| IBIS file 70t3519z.ibs created by s2ibis2 version 1.1
| North Carolina State University Electronics Research Laboratory  1995
[IBIS ver]   2.1
[File name]   70t3519bf.ibs
[File Rev]   3.0
|1.0 : Original Version - Wei-Ling Chang
|2.0 : Corrected Ramp rates and package RLC values - Wei-Ling Chang
|3.0 : Replaced I/O and Input models with ADC models - Sunil Kashyap
[Date]   03/30/04
[Disclaimer] Integrated Device Technology, Inc. ("IDT") hereby grants the
   user of this IBIS model a non-exclusive, nontransferable
   license to use this IBIS model under the following terms. The
   user is granted this license only to use the IBIS model and is
   not granted rights to sell, copy (except as needed to run the
   IBIS model), rent, lease or sub-license the IBIS model in
   whole or in part, or in modified form to anyone. The User may
   modify the IBIS model to suit its specific applications, but
   rights to derivative works and such modifications shall belong
   to IDT. This IBIS model is provided on an AS IS" basis and IDT
   makes absolutely no warranty with respect to the information
   contained herein. IDT DISCLAIMS AND CUSTOMER WAIVES ALL
   WARRANTIES, EXPRESS AND IMPLIED, INCLUDING WARRANTIES OF
   MERCHANTABILITY AND FITNESS FOR A PARTICULAR PURPOSE. THE
   ENTIRE RISK AS TO QUALITY AND PERFORMANCE IS WITH THE USER
   ACCORDINGLY, IN NO EVENT SHALL IDT BE LIABLE FOR ANY DIRECT OR
   INDIRECT DAMAGES, WHETHER IN CONTRACT OR TORT, INCLUDING ANY
   LOST PROFITS OR OTHER INCIDENTAL, CONSEQUENTIAL, EXEMPLARY, OR
   PUNITIVE DAMAGES ARISING OUT OF THE USE OR APPLICATION OF THE
   IBIS model. Further, IDT reserves the right to make changes
   without notice to any product herein to improve reliability,
   function, or design. IDT does not convey any license under
   patent rights or any other intellectual property rights,
   including those of third parties. IDT is not obligated to
   provide maintenance or support for the licensed IBIS model.
[Copyright]   Copyright 2001, Integrated Device Technology, Inc. all rights
   reserved
|   Component 70t3519z
[Component]   70t3519z
[Manufacturer]   Integrated Device Technology
[Package]
|208-pin fpBGA
| variable   typ   min   max
R_pkg   0.10000   0.05000   0.30000
L_pkg   12.0000nH   10.0000nH   14.00000nH
C_pkg   2.80000pF   1.50000pF   6.00000pF
| NOTE:
| The model_name inpad25, inpadzz25, inpadbs25, and iopad25 work for both
| 3.3v and 2.5v vddq.  When vddq is 3.3v, the model names are inpad33,
| inpadzz33, inpadbs33, and iopad33.  When vddq is 2.5v, the model names
| will be inpad25, inpadzz25, inpadbs25, and iopad25.
[Pin]  signal_name   model_name   R_pin   L_pin   C_pin
A1   io19l   iopad25
C2   io19r   iopad25
D4   io20l   iopad25
B1   io20r   iopad25
C1   vddql   POWER
A3   vss/test   GND
D3   io21l   iopad25
E4   io21r   iopad25
D1   io22l   iopad25
E2   io22r   iopad25
C3   vddqr   POWER
A17   vss   GND
E1   io23l   iopad25
F2   io23r   iopad25
F3   io24l   iopad25
G4   io24r   iopad25
F1   vddql   POWER
B2   vss   GND
G3   io25l   iopad25
H4   io25r   iopad25
G1   io26l   iopad25
H2   io26r   iopad25
E3   vddqr   POWER
B10   vss   GND
H1   vdd   POWER
J2   vdd   POWER
C10   vss   GND
J1   vddql   POWER
J4   zzr   inpadzz25
K3   io27r   iopad25
L4   io27l   iopad25
K1   io28r   iopad25
L2   io28l   iopad25
H3   vddqr   POWER
C17   vss   GND
L1   io29r   iopad25
M2   io29l   iopad25
M3   io30r   iopad25
N4   io30l   iopad25
M1   vddql   POWER
D2   vss   GND
N3   io31r   iopad25
N1   io31l   iopad25
P1   io32r   iopad25
P2   io32l   iopad25
L3   vddqr   POWER
E16   vss   GND
T1   io33r   iopad25
R2   io33l   iopad25
R3   io34r   iopad25
T2   io34l   iopad25
F4   vss   GND
T3   vddql   POWER
P4   io35r   iopad25
U2   io35l   iopad25
U3   plftr#   inpad25
U4   colr#   iopad25
T4   tms   inpadbs25
R4   tck   inpadbs25
P5   trstb   inpadbs25
T5   intr#   iopad25
R5   a17r   inpad25
P6   a16r   inpad25
U5   a15r   inpad25
T6   a14r   inpad25
R6   a13r   inpad25
P7   a12r   inpad25
U6   a11r   inpad25
T7   a10r   inpad25
R7   a9r   inpad25
P8   a8r   inpad25
U7   a7r   inpad25
T8   be3rb   inpad25
R8   be2rb   inpad25
P9   be1rb   inpad25
U8   be0rb   inpad25
T9   ce1r   inpad25
R9   ce0r   inpad25
C4   plftl#   inpad25
D9   vdd   POWER
F14   vss   GND
G2   vss   GND
P11   clkr#   inpad25
U10   oerb   inpad25
T11   rwrb   inpad25
R11   adsr#   inpad25
P12   cntenr#   inpad25
U11   repeatr#   inpad25
T12   a6r   inpad25
R12   a5r   inpad25
P13   a4r   inpad25
U12   a3r   inpad25
T13   a2r   inpad25
R13   a1r   inpad25
U13   a0r   inpad25
U9   vdd   POWER
H16   vss   GND
J3   vss   GND
U15   optr   inpad25
U16   io0l   iopad25
T15   io0r   iopad25
R15   vddql   POWER
J16   vss   GND
U17   io1l   iopad25
R16   io1r   iopad25
P14   io2l   iopad25
T17   io2r   iopad25
P3   vddqr   POWER
K2   vss   GND
P15   io3l   iopad25
N14   io3r   iopad25
P17   io4l   iopad25
N16   io4r   iopad25
N15   vddql   POWER
K4   vss   GND
N17   io5l   iopad25
M16   io5r   iopad25
M15   io6l   iopad25
L14   io6r   iopad25
R17   vddqr   POWER
K17   vss   GND
L15   io7l   iopad25
K14   io7r   iopad25
L17   io8l   iopad25
K16   io8r   iopad25
K15   vddql   POWER
L16   vss   GND
M4   vss   GND
M14   vss   GND
A10   vdd   POWER
P10   vdd   POWER
M17   vddqr   POWER
N2   vss   GND
H15   io9r   iopad25
G14   io9l   iopad25
H17   io10r   iopad25
G16   io10l   iopad25
G15   vddql   POWER
P16   vss   GND
G17   io11r   iopad25
F16   io11l   iopad25
F15   io12r   iopad25
E14   io12l   iopad25
J17   vddqr   POWER
R1   vss   GND
E15   io13r   iopad25
E17   io13l   iopad25
D17   io14r   iopad25
D16   io14l   iopad25
D15   vddql   POWER
J14   zzl   inpadzz25
B17   io15r   iopad25
C16   io15l   iopad25
C15   io16r   iopad25
B16   io16l   iopad25
R10   vss   GND
F17   vddqr   POWER
D14   io17r   iopad25
A16   io17l   iopad25
A15   optl   inpad25
D13   vdd   POWER
C14   vdd   POWER
A14   a0l   inpad25
B13   a1l   inpad25
C13   a2l   inpad25
D12   a3l   inpad25
A13   a4l   inpad25
B12   a5l   inpad25
C12   a6l   inpad25
A12   cntenl#   inpad25
B11   adsl#   inpad25
C11   rwlb   inpad25
D10   oelb   inpad25
A11   clkl   inpad25
T10   vss   GND
T14   vss   GND
H14   vdd   POWER
U14   vdd   POWER
B9   ce0lb   inpad25
C9   ce1l   inpad25
D8   be0lb   inpad25
A9   be1lb   inpad25
B8   be2lb   inpad25
C8   be3lb   inpad25
D7   a7l   inpad25
A8   a8l   inpad25
B7   a9l   inpad25
C7   a10l   inpad25
D6   a11l   inpad25
A7   a12l   inpad25
B6   a13l   inpad25
C6   a14l   inpad25
D5   a15l   inpad25
A6   a16l   inpad25
B5   a17l   inpad25
C5   intl#   iopad25
A4   tdo   iopad25
B4   tdi   inpadbs25
J15   vdd   POWER
T16   vss   GND
A2   io18l   iopad25
B3   io18r   iopad25
B15   vddqr   POWER
U1   vss   GND
A5   coll#   iopad25
D11   repeatl#   inpad25
|in   in   dummy_model
|oe   oe   dummy_model
| needed to give pads seperate POWER supply
[Pin Mapping] pulldown_ref   pullup_ref
A5   vss   vddql
A1   vss   vddql
C2   vss   vddqr
D4   vss   vddql
B1   vss   vddqr
C1   nc   vddql
A3   vss   nc
D3   vss   vddql
E4   vss   vddqr
D1   vss   vddql
E2   vss   vddqr
C3   nc   vdd
A17   vss   nc
E1   vss   vddql
F2   vss   vddqr
F3   vss   vddql
G4   vss   vddqr
F1   nc   vdd
B2   vss   nc
G3   vss   vddql
H4   vss   vddqr
G1   vss   vddql
H2   vss   vddqr
E3   nc   vddqr
B10   vss   nc
H1   nc   vdd
J2   nc   vdd
C10   vss   nc
J1   nc   vddql
J4   vss   vdd
K3   vss   vddqr
L4   vss   vddql
K1   vss   vddqr
L2   vss   vddql
H3   nc   vddqr
C17   vss   nc
L1   vss   vddqr
M2   vss   vddql
M3   vss   vddqr
N4   vss   vddql
M1   nc   vddql
D2   vss   nc
N3   vss   vddqr
N1   vss   vddql
P1   vss   vddqr
P2   vss   vddql
L3   nc   vddqr
E16   vss   nc
T1   vss   vddqr
R2   vss   vddql
R3   vss   vddqr
T2   vss   vddql
F4   vss   nc
T3   nc   vddql
P4   vss   vddqr
U2   vss   vddql
U3   vss   vddqr
U4   vss   vddqr
T4   vss   vdd
R4   vss   vdd
P5   vss   vdd
T5   vss   vddqr
R5   vss   vdd
P6   vss   vdd
U5   vss   vdd
T6   vss   vdd
R6   vss   vdd
P7   vss   vdd
U6   vss   vdd
T7   vss   vdd
R7   vss   vdd
P8   vss   vdd
U7   vss   vdd
T8   vss   vdd
R8   vss   vdd
P9   vss   vdd
U8   vss   vdd
T9   vss   vdd
R9   vss   vdd
C4   vss   vddql
D9   nc   vdd
F14   vss   nc
G2   vss   nc
P11   vss   vddqr
U10   vss   vdd
T11   vss   vdd
R11   vss   vddqr
P12   vss   vddqr
U11   vss   vddqr
T12   vss   vdd
R12   vss   vdd
P13   vss   vdd
U12   vss   vdd
T13   vss   vdd
R13   vss   vdd
U13   vss   vdd
U9   nc   vdd
H16   vss   nc
J3   vss   nc
U15   vss   vdd
U16   vss   vddql
T15   vss   vddqr
R15   nc   vddql
J16   vss   nc
U17   vss   vddql
R16   vss   vddqr
P14   vss   vddql
T17   vss   vddqr
P3   nc   vddqr
K2   vss   nc
P15   vss   vddql
N14   vss   vddqr
P17   vss   vddql
N16   vss   vddqr
N15   nc   vddql
K4   vss   nc
N17   vss   vddql
M16   vss   vddqr
M15   vss   vddql
L14   vss   vddqr
R17   nc   vddqr
K17   vss   nc
L15   vss   vddql
K14   vss   vddqr
L17   vss   vddql
K16   vss   vddqr
K15   nc   vddql
L16   vss   nc
M4   vss   nc
M14   vss   nc
A10   nc   vdd
P10   nc   vdd
M17   nc   vddqr
N2   vss   nc
H15   vss   vddqr
G14   vss   vddql
H17   vss   vddqr
G16   vss   vddql
G15   nc   vddql
P16   vss   nc
G17   vss   vddqr
F16   vss   vddql
F15   vss   vddqr
E14   vss   vddql
J17   nc   vddqr
R1   vss   nc
E15   vss   vddqr
E17   vss   vddql
D17   vss   vddqr
D16   vss   vddql
D15   nc   vdd
J14   vss   vdd
B17   vss   vddqr
C16   vss   vddql
C15   vss   vddqr
B16   vss   vddql
R10   vss   nc
F17   nc   vddqr
D14   vss   vddqr
A16   vss   vddql
A15   vss   vdd
D13   nc   vdd
C14   nc   vdd
A14   vss   vdd
B13   vss   vdd
C13   vss   vdd
D12   vss   vdd
A13   vss   vdd
B12   vss   vdd
C12   vss   vdd
A12   vss   vddql
B11   vss   vddql
C11   vss   vdd
D10   vss   vdd
D11   vss   vddql
A11   vss   vddql
T10   vss   nc
T14   vss   nc
H14   nc   vdd
U14   nc   vdd
B9   vss   vdd
C9   vss   vdd
D8   vss   vdd
A9   vss   vdd
B8   vss   vdd
C8   vss   vdd
D7   vss   vdd
A8   vss   vdd
B7   vss   vdd
C7   vss   vdd
D6   vss   vdd
A7   vss   vdd
B6   vss   vdd
C6   vss   vdd
D5   vss   vdd
A6   vss   vdd
B5   vss   vdd
C5   vss   vddql
A4   vss   vdd
B4   vss   vdd
J15   nc   vdd
T16   vss   nc
A2   vss   vddql
B3   vss   vddqr
B15   nc   vddqr
U1   vss   nc
| Models and submodels in the file (8): inpad25 (Input), inpad33 (Input), inpadzz25 (Input), inpadzz33 (Input), inpadbs25 (Input), inpadbs33 (Input), iopad25 (I/O), iopad33 (I/O)
